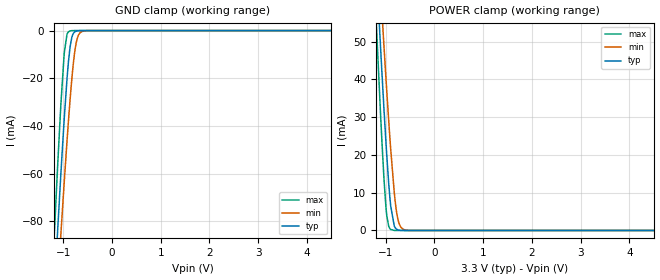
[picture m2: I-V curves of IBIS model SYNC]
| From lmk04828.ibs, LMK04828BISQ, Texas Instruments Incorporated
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|   Model   SYNC
[Model]   SYNC
Model_type   Input
Vinl = 0.4
Vinh = 1.2
|   typ   min   max
|   (nom PVT)   (fast PVT)   (slow PVT)
C_comp   0.1841pF   0.1807pF   0.1863pF
[Voltage Range]   3.3   3.15   3.45
[Temperature Range]   27   125   -40
[Power Clamp Reference]   3.3   3.15   3.45
[GND Clamp Reference]   0   0   0
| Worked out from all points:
|   GND clamp passes 1 mA (typ) near -0.79 V on its own axis
|   POWER clamp passes 1 mA (typ) near -0.82 V on its own axis
[GND Clamp]
|   Voltage   I(typ)   I(min)   I(max)
-3.3V     -965.6mA   -893.6mA   -1.069A
-1.191V   -112.1mA   -132.7mA   -88.59mA
-1.117V   -84.4mA    -107.7mA   -57.4mA
-1.048V   -59.55mA   -84.92mA   -30.5mA
-978.5mV  -36.37mA   -62.95mA   -9.221mA
-924mV    -20.4mA    -46.56mA   -1.598mA
-859.7mV  -6.75mA    -28.81mA   -125.9uA
-795.3mV  -1.278mA   -14.16mA   -6.167uA
-735.9mV  -231.4uA   -5.307mA   -320.6nA
-681.5mV  -39.54uA   -1.674mA   -17.85nA
-577.5mV  -941.8nA   -148.2uA   0A
6.595V    0A         0A         0A
[POWER Clamp]
|   Voltage   I(typ)   I(min)   I(max)
-3.3V     638.8mA    590.5mA    708.3mA
-1.196V   70.39mA    83.75mA    55.37mA
-1.107V   48.47mA    63.9mA     30.8mA
-1.077V   41.42mA    57.43mA    23.19mA
-1.038V   32.31mA    48.95mA    13.93mA
-978.5mV  19.65mA    36.67mA    3.829mA
-899.2mV  6.493mA    21.57mA    264.8uA
-825mV    1.174mA    9.968mA    10.77uA
-765.6mV  254.2uA    3.922mA    572nA
-701.3mV  35.15uA    1.11mA     20.08nA
-582.5mV  493.7nA    81.77uA    0A
6.595V    0A         0A         0A
